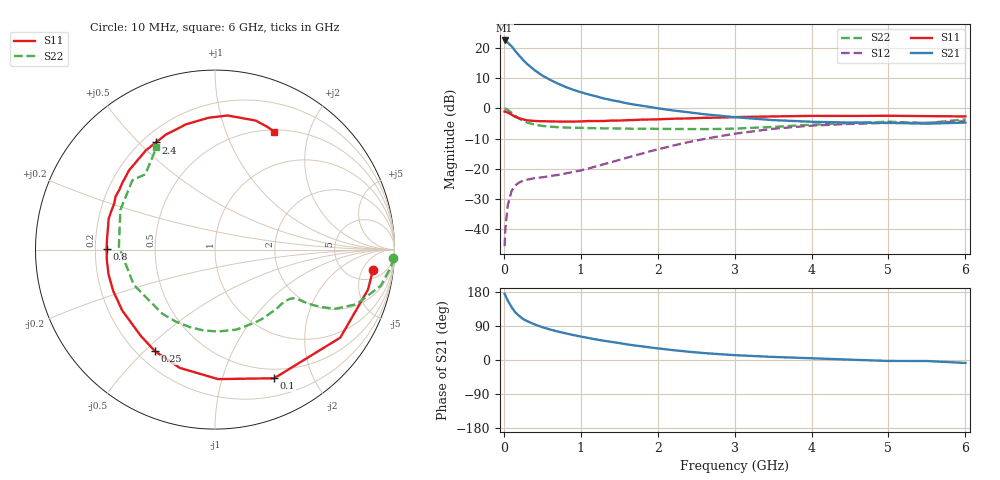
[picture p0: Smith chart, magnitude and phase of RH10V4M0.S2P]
! SIEMENS Small Signal Semiconductors
! BFR106
! Si NPN RF Bipolar Junction Transistor in SOT23
! VCE = 10 V  IC = 4 mA
! Common Emitter S-Parameters:  August  1996
# GHz  S  MA  R  50
!  f  S11  S21  S12  S22
! GHz  MAG  ANG  MAG  ANG  MAG  ANG  MAG  ANG
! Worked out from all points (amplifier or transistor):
!   36 points, 10 MHz to 6 GHz, reference 50 ohm
!   highest |S21| = 22.4 dB at 10 MHz (marker M1)
!   |S21| within 3 dB of that: start of sweep to 133.5 MHz
!   unconditionally stable (mu >= 1): 675.3 MHz to 1.822 GHz; 4.886 GHz to end of sweep
!   at 250 MHz: K = 0.44, MSG = 19.9 dB, |S12| = -23.9 dB
!   at 1.4 GHz: K = 1.15, MAG = 7.9 dB, |S12| = -17.8 dB
!   at 6 GHz: K = 1.02, MAG = -1.1 dB, |S12| = -4.3 dB
!   S11 on the Smith chart (normalised r, x): 10 MHz: 8, -8; 100 MHz: 0.39, -1.49; 250 MHz: 0.27, -0.54; 800 MHz: 0.25, +0.00; 2.4 GHz: 0.25, +0.56; 6 GHz: 0.52, +1.49
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0.01  0.8876 -7.3  13.2 174.6  0.0053 88.4  0.9947 -2.7
0.02  0.881 -14.7  13.05 170.8  0.0102 83.4  0.987 -5.3
0.05  0.8531 -35.1  12.18 157.1  0.0247 71.8  0.9455 -12.3
0.1  0.7891 -65.3  10.6 139.8  0.0431 58.6  0.8454 -21.1
0.15  0.7217 -88.7  8.783 125.5  0.0535 48.0  0.7466 -26.2
0.2  0.6877 -106.6  7.418 116.2  0.0597 43.2  0.6758 -28.3
0.25  0.6575 -120.5  6.307 108.2  0.0639 39.6  0.6198 -29.7
0.3  0.6344 -130.6  5.442 102.8  0.0663 38.5  0.5842 -30.3
0.4  0.6182 -146.7  4.265 93.9  0.0703 37.6  0.538 -30.9
0.5  0.6123 -157.8  3.475 86.6  0.0726 38.8  0.5128 -31.9
0.6  0.6092 -166.8  2.963 80.6  0.0763 41.4  0.4984 -33.5
0.8  0.6039 179.8  2.265 70.6  0.084 47.7  0.4812 -37.8
1.1  0.617 163.9  1.698 58.0  0.1016 57.5  0.4725 -46.1
1.3  0.6173 155.5  1.457 50.8  0.1197 62.5  0.4674 -52.5
1.6  0.6365 144.2  1.211 41.3  0.1527 66.7  0.462 -63.2
2.2  0.6736 124.9  0.922 26.0  0.2424 65.9  0.4567 -88.2
2.4  0.6815 118.8  0.861 21.9  0.277 63.7  0.4548 -98.4
3.5  0.7354 92.8  0.639 8.1  0.46 43.4  0.4933 -156.5
4.5  0.7482 78.0  0.582 0.9  0.5533 22.1  0.5716 157.3
5  0.7538 72.5  0.576 -2.5  0.574 13.3  0.6012 139.9
5.5  0.7436 67.0  0.558 -2.7  0.5766 8.8  0.5715 132.8
6  0.7358 63.3  0.581 -7.8  0.6111 0.4  0.6564 119.8
